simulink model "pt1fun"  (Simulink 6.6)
settings: Solver=ode45  StartTime=0.0  StopTime=10.0  RelTol=1e-3

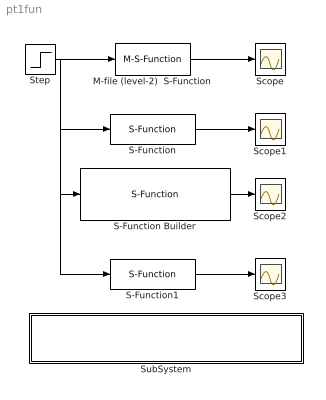
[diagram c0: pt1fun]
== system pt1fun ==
  M-file (level-2)  S-Function : M-S-Function  FunctionName=pt1sfun_m2  Parameters=T
  S-Function : S-Function  FunctionName=pt1sfun_c  Parameters=T
  S-Function Builder : S-Function  FunctionName=pt1sfun_csfb  Parameters=T  SFunctionModules=pt1sfun_csfb_wrapper  WizardData=DataTag0
  S-Function1 : S-Function  FunctionName=pt1sfun_m  Parameters=T
  Scope{,1..3} (4 alike) : Scope
  Step : Step  SampleTime=0
  SubSystem : Subsystem
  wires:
  Step/1 -> S-Function/1, S-Function1/1, S-Function Builder/1, M-file (level-2)  S-Function/1
  M-file (level-2)  S-Function/1 -> Scope/1
  S-Function/1 -> Scope1/1
  S-Function1/1 -> Scope3/1
  S-Function Builder/1 -> Scope2/1

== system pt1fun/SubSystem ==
